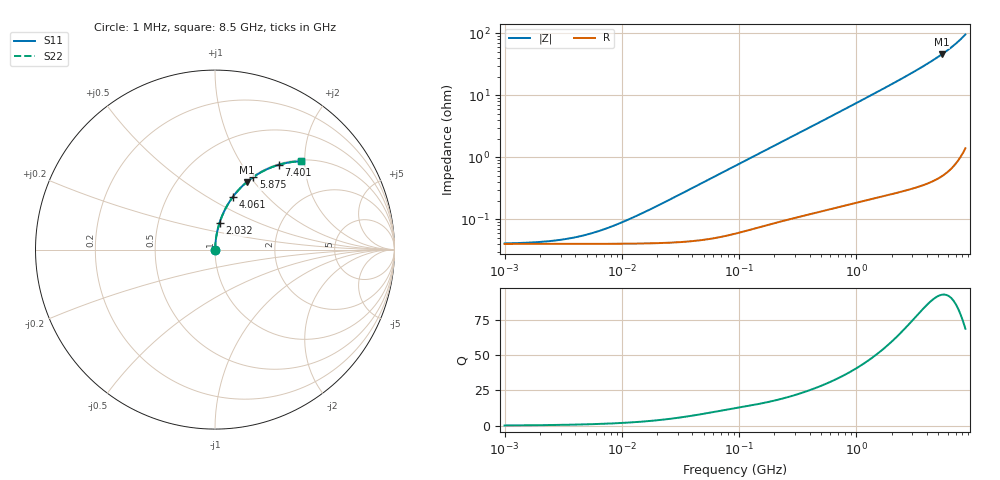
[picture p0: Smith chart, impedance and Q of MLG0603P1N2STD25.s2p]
! S-Parameter Data Generated by TDK Corporation
! Copyright(C) 2025 TDK Corporation.
! All Rights Reserved.
! TDK P/N: MLG0603P1N2STD25 (SMD / SMT Inductor (Coil))
! Property: L=1.2nH at 500MHz
! Size(LxWxT): 0.6x0.3x0.3mm
! Model Type: s2p (Touchstone File Format Version 1.0)
! Frequency: DC=Yes Start=1MHz Stop=8500MHz 198points Log-sweep
! Model Generated on Feb. 6, 2025
! Terms and conditions regarding TDK Simulation Models:
! 1)This simulation model is being provided solely for informational
!  purposes. Please refer to the specifications of the products in
!  terms of detailed characteristics of such products.
! 2)In no event shall TDK Corporation of any of its subsidiaries be
!  liable for any loss or damage arising, directly or indirectly,
!  from any information contained in this simulation model, including,
!  but not limited to loss or damages arising from any inaccuracies,
!  omissions or errors in connection with such information.
! 3)Any and all copyrights on this simulation model are owned by
!  TDK Corporation.  Duplication or redistribution of this simulation
!  model without prior written permission from TDK Corporation
!  is prohibited.
! 4)This simulation model is subject to any modification or change
!  without any prior notice.
! 5)Neither TDK Corporation nor any of its subsidiaries shall make any
!  warranty, express or implied, including but not limited to the
!  correctness, implied warranties of merchantability and fitness for
!  a particular purpose with respect to this simulation models.
! 6)The use of this simulation model shall be deemed to have consented
!  to the terms and conditions hereof.
! Port Assignments:
!  1 ---@@@--- 2
! Applicable Conditions:
!  Temperature = 25 degC
!  DC Bias Current = 0 A
!  Small Signal Operation
# Hz S MA R 50
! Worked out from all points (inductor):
!   197 points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, 1 MHz to 8.5 GHz, reference 50 ohm
!   read as one part in series: L = 1.26 nH near 15.95 MHz
!   highest Q = 92.6 at 5.357 GHz (marker M1), where L = 1.36 nH
!   S11 on the Smith chart (normalised r, x): 1 MHz: 1.00, +0.00; 2.032 GHz: 1.01, +0.31; 4.061 GHz: 1.01, +0.65; 5.875 GHz: 1.01, +1.04; 7.401 GHz: 1.02, +1.48; 8.5 GHz: 1.03, +1.91
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1000000  0.0004077 11.2  0.9996 -0.0  0.9996 -0.0  0.0004077 11.2
1661608  0.0004212 18.3  0.9996 -0.0  0.9996 -0.0  0.0004212 18.3
2403882  0.0004433 25.5  0.9996 -0.0  0.9996 -0.0  0.0004433 25.5
3320851  0.0004793 33.4  0.9996 -0.0  0.9996 -0.0  0.0004793 33.4
4587603  0.0005415 42.3  0.9996 -0.0  0.9996 -0.0  0.0005415 42.3
6337562  0.0006437 51.4  0.9996 -0.0  0.9996 -0.0  0.0006437 51.4
8755050  0.0008034 59.9  0.9996 -0.0  0.9996 -0.0  0.0008034 59.9
1.26661e7  0.001084 68.0  0.9996 -0.1  0.9996 -0.1  0.001084 68.0
2.10461e7  0.001721 76.0  0.9996 -0.1  0.9996 -0.1  0.001721 76.0
9.219544e7  0.007242 85.0  0.9994 -0.4  0.9994 -0.4  0.007242 85.0
4.229561e8  0.03194 86.0  0.9983 -1.8  0.9983 -1.8  0.03194 86.0
1.016736e9  0.07584 84.3  0.9953 -4.3  0.9953 -4.3  0.07584 84.3
1.940355e9  0.1445 80.7  0.987 -8.3  0.987 -8.3  0.1445 80.7
2.032026e9  0.1514 80.3  0.986 -8.7  0.986 -8.7  0.1514 80.3
2.939772e9  0.2203 76.5  0.9724 -12.7  0.9724 -12.7  0.2203 76.5
4.061159e9  0.3082 71.4  0.9478 -17.9  0.9478 -17.9  0.3082 71.4
4.664383e9  0.3569 68.5  0.9302 -20.9  0.9302 -20.9  0.3569 68.5
5.357206e9  0.4143 64.9  0.9057 -24.5  0.9057 -24.5  0.4143 64.9
5.87536e9  0.4581 62.1  0.8839 -27.3  0.8839 -27.3  0.4581 62.1
6.748056e9  0.5334 57.1  0.8398 -32.2  0.8398 -32.2  0.5334 57.1
7.400733e9  0.5904 53.1  0.8 -36.2  0.8 -36.2  0.5904 53.1
8.5e9  0.6859 45.9  0.7177 -43.3  0.7177 -43.3  0.6859 45.9
